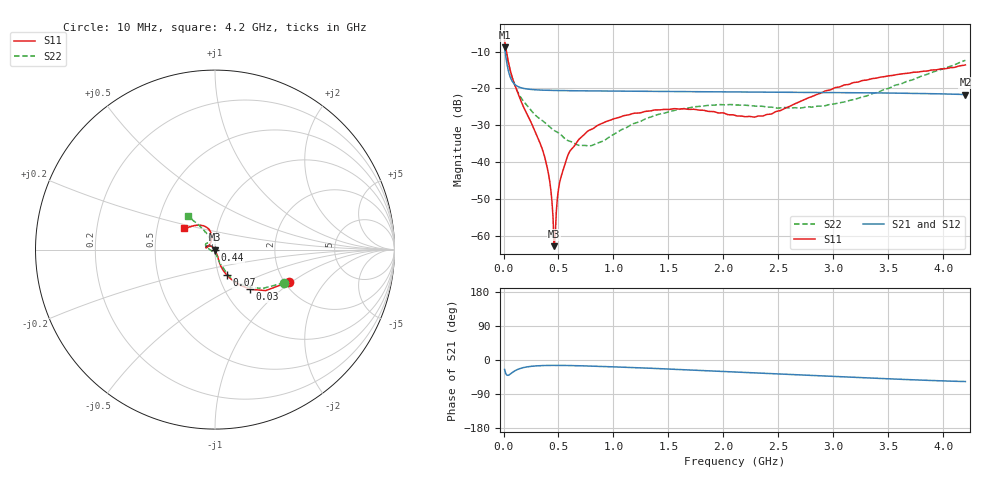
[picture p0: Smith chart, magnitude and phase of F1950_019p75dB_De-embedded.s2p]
! Integrated Device Technology
! Corporate Headquarters
! 6024 Silver Creek Valley Road
! San Jose, CA 95138  USA
! Phone:  1-408-284-8200
! Toll Free:  1-800-223-1366
! Webpage:  http://www.idt.com/
! Timing and RF Division
! 515 Groton Road, Suite 102
! Westford, MA 01886-6024
! Device:  F1950
! Description: 7-bit 0.25 dB Digital Step Attenuator
! Frequency:  150.0 -  4000.00 MHz
! Package:  4x4 mm Thin QFN Plastic Package: 24 pin
! Ports:  2 RF, 12 DC
!  Pin  1  = D0
!  Pin  2  = VDD
!  Pin  3  = Vmode
!  Pin  4  = GND
!  Pin  5  = RF1  =  Port 1
!  Pin  6  = GND
!  Pin  7  = GND
!  Pin  8  = GND
!  Pin  9  = GND
!  Pin 10  = GND
!  Pin 11  = GND
!  Pin 12  = GND
!  Pin 13  = GND
!  Pin 14  = RF2  =  Port 2
!  Pin 15  = GND
!  Pin 16  = LE
!  Pin 17  = CLK
!  Pin 18  = DATE
!  Pin 19  = D6
!  Pin 20  = D5
!  Pin 21  = D4
!  Pin 22  = D3
!  Pin 23  = D2
!  Pin 24  = D1
! State:  79
! Atten State:  19.75 dB
! Voltage:  +5.00 Volts
! Current:  Not Measured mA
! Data:  The device was measured on a the F195X evaluation board which has
!  individual transmission lines to the RF pins.  Data was collected
!  using a calibrated network analyzer.  The evaluation board was
!  de-embedded using a TRL calibration technique.
!  The reference plane is the edge of the package pin.
! Misc:  Board 2019
!  Action Tracker AT0250
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# GHz S dB R 50
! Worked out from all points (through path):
!   420 points, 10 MHz to 4.2 GHz, reference 50 ohm
!   highest |S21| = -8.89 dB at 10 MHz (marker M1); lowest = -21.6 dB at 4.2 GHz (marker M2)
!   group delay of S21, straight-line fit = 29.3 ps
!   lowest |S11| = -62.8 dB at 460 MHz (marker M3), VSWR 1.00, Z = 50 - j0.0661 ohm
!   |S11| at or under -10 dB: 26.77 MHz to end of sweep
!   |S22| runs from -35.6 to -7.4 dB; largest |S21 - S12| = 0.00015
!   S11 on the Smith chart (normalised r, x): 10 MHz: 2.10, -0.95; 30 MHz: 1.31, -0.64; 70 MHz: 1.09, -0.32; 440 MHz: 1.00, -0.01; 4.2 GHz: 0.69, +0.17
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0.01  -6.98 -23.8  -8.89 -25.0  -8.89 -25.0  -7.38 -25.6
0.03  -10.58 -48.3  -13.07 -39.8  -13.07 -39.8  -11.01 -48.1
0.07  -16.06 -65.0  -17.54 -35.2  -17.54 -35.2  -16.16 -63.0
0.16  -23.50 -71.1  -19.81 -21.7  -19.81 -21.6  -22.54 -69.5
0.36  -37.17 -65.2  -20.46 -14.6  -20.46 -14.6  -28.87 -74.9
0.41  -43.33 -68.3  -20.50 -14.3  -20.50 -14.3  -30.13 -75.6
0.43  -47.47 -71.8  -20.52 -14.2  -20.52 -14.2  -30.66 -77.2
0.44  -50.41 -74.7  -20.53 -14.2  -20.53 -14.2  -30.94 -78.4
0.46  -62.78 -114.4  -20.54 -14.2  -20.54 -14.2  -31.37 -81.0
0.48  -53.56 136.0  -20.55 -14.2  -20.55 -14.2  -31.71 -83.2
0.51  -45.55 132.5  -20.57 -14.2  -20.57 -14.2  -32.23 -85.1
0.56  -40.38 130.5  -20.59 -14.4  -20.59 -14.4  -33.67 -89.9
0.61  -36.73 133.1  -20.61 -14.6  -20.61 -14.6  -34.36 -99.4
0.71  -33.13 135.4  -20.64 -15.3  -20.64 -15.3  -35.44 -117.6
0.81  -30.95 138.9  -20.67 -16.2  -20.67 -16.2  -35.39 -140.0
0.99  -28.37 145.9  -20.73 -18.0  -20.73 -18.0  -32.68 -169.0
1.41  -25.82 162.2  -20.83 -22.7  -20.83 -22.7  -27.03 166.1
2.11  -27.36 156.7  -20.95 -31.5  -20.94 -31.5  -24.47 147.5
2.43  -26.96 124.1  -21.00 -35.5  -21.00 -35.5  -25.06 137.4
2.81  -22.14 103.8  -21.06 -40.6  -21.06 -40.7  -25.04 122.2
3.51  -16.54 116.5  -21.24 -49.7  -21.23 -49.8  -19.89 117.4
4.2  -13.61 145.6  -21.64 -56.8  -21.64 -56.9  -12.37 129.0
